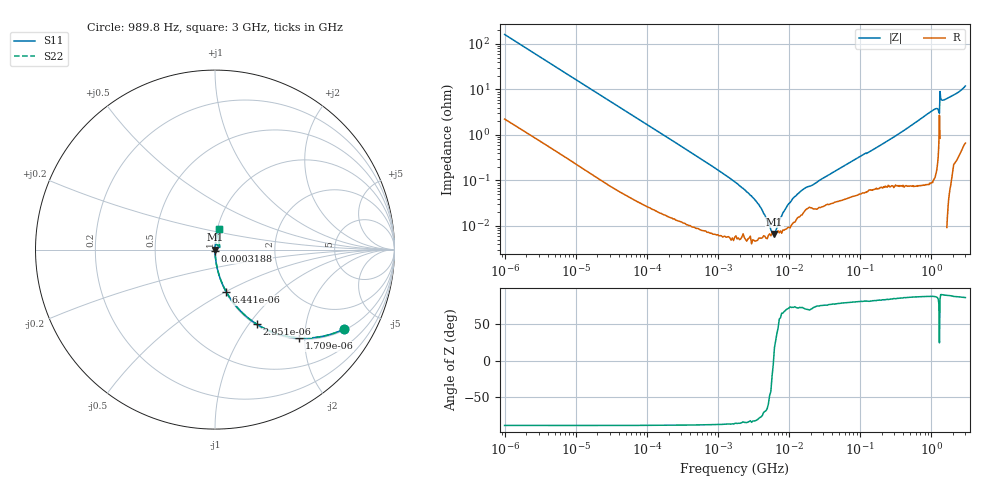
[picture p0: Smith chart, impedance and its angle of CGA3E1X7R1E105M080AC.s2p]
! S-Parameter Data Generated by TDK Corporation
! Copyright(C) 2020 TDK Corporation.
! All Rights Reserved.
! TDK P/N: CGA3E1X7R1E105M080AC (Multilayer Ceramic Chip Capacitor)
! Property: C=1uF
! Size(LxWxT): 1.6x0.8x0.8mm
! Model Type: s2p (Touchstone File Format Version 1.0)
! Frequency: DC=Yes Start=0.000989846MHz Stop=3000MHz 463points Log-sweep
! Model Generated on Aug. 18, 2020
! Port Assignments:
!  1 ---| |--- 2
! Applicable Conditions:
!  Temperature = 25 degC
!  DC Bias Voltage = 0 V
!  Small Signal Operation
! Terms and conditions regarding TDK Simulation Models
! (1)This simulation model is being provided solely for informational purposes. Please refer to the specifications of the products in terms of detailed characteristics of such products.
! (2)In no event shall TDK Corporation of any of its subsidiaries be liable for any loss or damage arising, directly or indirectly,
!  From any information contained in this simulation model, including, but not limited to loss or damages arising from any inaccuracies, omissions or errors in connection with such information.
! (3)Any and all copyrights on this simulation model are owned by TDK Corporation.
!  Duplication or redistribution of this simulation model without prior written permission from TDK Corporation is prohibited.
! (4)This simulation model is subject to any modification or change without any prior notice.
! (5)Neither TDK Corporation nor any of its subsidiaries shall make any warranty, express or implied,
!  Including but not limited to the correctness, implied warranties of merchantability and fitness for a particular purpose with respect to this simulation models.
! (6)The use of this simulation model shall be deemed to have consented to the terms and conditions hereof.
# Hz S MA R 50
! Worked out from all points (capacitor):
!   462 points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, 989.8 Hz to 3 GHz, reference 50 ohm
!   read as one part in series: C = 994 nF near 1.07 kHz
!   lowest |Z| = 6.7 mohm at 6.185 MHz (marker M1)
!   series resonance near 6.007 MHz, so ESL is about 710 pH
!   S11 on the Smith chart (normalised r, x): 989.8 Hz: 1.04, -3.23; 1.709 kHz: 1.03, -1.88; 2.951 kHz: 1.02, -1.09; 6.441 kHz: 1.01, -0.50; 318.8 kHz: 1.00, -0.01; 3 GHz: 1.01, +0.24
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989.846  0.845 -31.5  0.5232 57.7  0.5232 57.7  0.845 -31.5
1709.24  0.6797 -46.4  0.724 42.8  0.724 42.8  0.6797 -46.4
2951.47  0.4765 -60.7  0.8725 28.5  0.8725 28.5  0.4765 -60.7
6440.891  0.244 -75.1  0.9663 14.1  0.9663 14.1  0.244 -75.1
12024.64  0.1351 -81.4  0.989 7.8  0.989 7.8  0.1351 -81.4
146075.1  0.01163 -88.4  0.9997 0.7  0.9997 0.7  0.01163 -88.4
318774.6  0.00536 -88.4  0.9999 0.3  0.9999 0.3  0.00536 -88.4
1774518  0.0008923 -86.0  0.9999 0.1  0.9999 0.1  0.0008923 -86.0
3186112  0.0003993 -83.0  1 0.0  1 0.0  0.0003993 -83.0
3872469  0.0002659 -78.2  0.9999 0.0  0.9999 0.0  0.0002659 -78.2
5291161  0.0001009 -48.1  0.9999 0.0  0.9999 0.0  0.0001009 -48.1
6184898  6.696e-05 17.9  0.9999 -0.0  0.9999 -0.0  6.696e-05 17.9
6952943  0.0001104 44.8  0.9999 -0.0  0.9999 -0.0  0.0001104 44.8
8787006  0.0002349 68.9  0.9999 -0.0  0.9999 -0.0  0.0002349 68.9
1.200615e7  0.0004454 74.2  0.9999 -0.0  0.9999 -0.0  0.0004454 74.2
2.073191e7  0.0007803 71.3  0.9998 -0.0  0.9998 -0.0  0.0007803 71.3
2.507343e8  0.0077 83.8  0.9992 -0.4  0.9992 -0.4  0.0077 83.8
1.059487e9  0.03528 86.4  0.9984 -2.0  0.9984 -2.0  0.03528 86.4
1.243477e9  0.03607 82.7  0.996 -2.1  0.996 -2.1  0.03607 82.7
1.374365e9  0.05984 87.5  0.9992 -3.4  0.9992 -3.4  0.05984 87.5
1.581072e9  0.06094 86.6  0.9982 -3.5  0.9982 -3.5  0.06094 86.6
3e9  0.1177 80.1  0.9865 -6.7  0.9865 -6.7  0.1177 80.1
